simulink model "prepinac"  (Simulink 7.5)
settings: Solver=ode45  StartTime=0.0  StopTime=20  FixedStep=1  MaxStep=1  RelTol=1e-3
libraries: commutil2 x32, dspmtrx3 x28, simulink x20
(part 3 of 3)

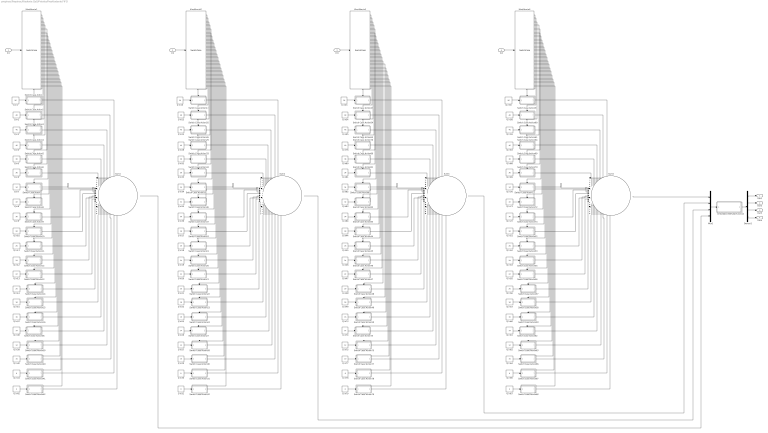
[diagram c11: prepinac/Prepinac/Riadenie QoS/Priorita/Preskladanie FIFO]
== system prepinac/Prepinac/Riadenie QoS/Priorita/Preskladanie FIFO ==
  In1 : Inport  OutDataType=sfix(16)  OutScaling=2^0
  In2 : Inport  Port=2  OutDataType=sfix(16)  OutScaling=2^0
  In3 : Inport  Port=3  OutDataType=sfix(16)  OutScaling=2^0
  In4 : Inport  Port=4  OutDataType=sfix(16)  OutScaling=2^0
  "     Embedded MATLAB Function" : Stateflow chart  TreatAsAtomicUnit=on
  Demux1 : Demux
  Klasifikacia{1..4} (4 alike) : SwitchCase  CaseConditions={0,8,10,12,14,16,18,20,22,24,26,28,30,32,34,36,38,40,46,48,56}  ShowDefaultCase=off
  Mux1 : Mux
  Q in{1,16,43,50} (4 alike) : Constant  Value=56  VectorParams1D=off  OutDataTypeMode=double  OutDataType=sfix(16)  OutScaling=2^0  OutDataTypeStr=double  SampleTime=-1
  Q in{10,17,44,51} (4 alike) : Constant  Value=28  VectorParams1D=off  OutDataTypeMode=double  OutDataType=sfix(16)  OutScaling=2^0  OutDataTypeStr=double  SampleTime=-1
  Q in{11,18,45,52} (4 alike) : Constant  Value=26  VectorParams1D=off  OutDataTypeMode=double  OutDataType=sfix(16)  OutScaling=2^0  OutDataTypeStr=double  SampleTime=-1
  Q in{12,19,46,53} (4 alike) : Constant  Value=24  VectorParams1D=off  OutDataTypeMode=double  OutDataType=sfix(16)  OutScaling=2^0  OutDataTypeStr=double  SampleTime=-1
  Q in{13,20,47,55} (4 alike) : Constant  Value=22  VectorParams1D=off  OutDataTypeMode=double  OutDataType=sfix(16)  OutScaling=2^0  OutDataTypeStr=double  SampleTime=-1
  Q in{14,21,48,56} (4 alike) : Constant  Value=20  VectorParams1D=off  OutDataTypeMode=double  OutDataType=sfix(16)  OutScaling=2^0  OutDataTypeStr=double  SampleTime=-1
  Q in{15,22,49,57} (4 alike) : Constant  Value=18  VectorParams1D=off  OutDataTypeMode=double  OutDataType=sfix(16)  OutScaling=2^0  OutDataTypeStr=double  SampleTime=-1
  Q in{2,23,54,58} (4 alike) : Constant  Value=48  VectorParams1D=off  OutDataTypeMode=double  OutDataType=sfix(16)  OutScaling=2^0  OutDataTypeStr=double  SampleTime=-1
  Q in{3,24,59,65} (4 alike) : Constant  Value=46  VectorParams1D=off  OutDataTypeMode=double  OutDataType=sfix(16)  OutScaling=2^0  OutDataTypeStr=double  SampleTime=-1
  Q in{25,37,60,73} (4 alike) : Constant  Value=16  VectorParams1D=off  OutDataTypeMode=double  OutDataType=sfix(16)  OutScaling=2^0  OutDataTypeStr=double  SampleTime=-1
  Q in{26,38,61,74} (4 alike) : Constant  Value=14  VectorParams1D=off  OutDataTypeMode=double  OutDataType=sfix(16)  OutScaling=2^0  OutDataTypeStr=double  SampleTime=-1
  Q in{27,39,62,75} (4 alike) : Constant  Value=12  VectorParams1D=off  OutDataTypeMode=double  OutDataType=sfix(16)  OutScaling=2^0  OutDataTypeStr=double  SampleTime=-1
  Q in{4,28,63,76} (4 alike) : Constant  Value=40  VectorParams1D=off  OutDataTypeMode=double  OutDataType=sfix(16)  OutScaling=2^0  OutDataTypeStr=double  SampleTime=-1
  Q in{29,40,64,77} (4 alike) : Constant  Value=10  VectorParams1D=off  OutDataTypeMode=double  OutDataType=sfix(16)  OutScaling=2^0  OutDataTypeStr=double  SampleTime=-1
  Q in{30,41,66,78} (4 alike) : Constant  Value=8  VectorParams1D=off  OutDataTypeMode=double  OutDataType=sfix(16)  OutScaling=2^0  OutDataTypeStr=double  SampleTime=-1
  Q in{31,42,67,79} (4 alike) : Constant  Value=0  VectorParams1D=off  OutDataTypeMode=double  OutDataType=sfix(16)  OutScaling=2^0  OutDataTypeStr=double  SampleTime=-1
  Q in{5,32,68,80} (4 alike) : Constant  Value=38  VectorParams1D=off  OutDataTypeMode=double  OutDataType=sfix(16)  OutScaling=2^0  OutDataTypeStr=double  SampleTime=-1
  Q in{6,33,69,81} (4 alike) : Constant  Value=36  VectorParams1D=off  OutDataTypeMode=double  OutDataType=sfix(16)  OutScaling=2^0  OutDataTypeStr=double  SampleTime=-1
  Q in{7,34,70,82} (4 alike) : Constant  Value=34  VectorParams1D=off  OutDataTypeMode=double  OutDataType=sfix(16)  OutScaling=2^0  OutDataTypeStr=double  SampleTime=-1
  Q in{8,35,71,83} (4 alike) : Constant  Value=32  VectorParams1D=off  OutDataTypeMode=double  OutDataType=sfix(16)  OutScaling=2^0  OutDataTypeStr=double  SampleTime=-1
  Q in{9,36,72,84} (4 alike) : Constant  Value=30  VectorParams1D=off  OutDataTypeMode=double  OutDataType=sfix(16)  OutScaling=2^0  OutDataTypeStr=double  SampleTime=-1
  Sum{1..4} (4 alike) : Sum  Inputs=|+++++++++++++++++++++  OutDataType=sfix(16)  OutScaling=2^0
  Switch Case Action1 : Subsystem  TreatAsAtomicUnit=on
  Switch Case Action10 : Subsystem  TreatAsAtomicUnit=on
  Switch Case Action11 : Subsystem  TreatAsAtomicUnit=on
  Switch Case Action12 : Subsystem  TreatAsAtomicUnit=on
  Switch Case Action13 : Subsystem  TreatAsAtomicUnit=on
  Switch Case Action14 : Subsystem  TreatAsAtomicUnit=on
  Switch Case Action15 : Subsystem  TreatAsAtomicUnit=on
  Switch Case Action16 : Subsystem  TreatAsAtomicUnit=on
  Switch Case Action17 : Subsystem  TreatAsAtomicUnit=on
  Switch Case Action18 : Subsystem  TreatAsAtomicUnit=on
  Switch Case Action19 : Subsystem  TreatAsAtomicUnit=on
  Switch Case Action2 : Subsystem  TreatAsAtomicUnit=on
  Switch Case Action20 : Subsystem  TreatAsAtomicUnit=on
  Switch Case Action21 : Subsystem  TreatAsAtomicUnit=on
  Switch Case Action22 : Subsystem  TreatAsAtomicUnit=on
  Switch Case Action23 : Subsystem  TreatAsAtomicUnit=on
  Switch Case Action24 : Subsystem  TreatAsAtomicUnit=on
  Switch Case Action25 : Subsystem  TreatAsAtomicUnit=on
  Switch Case Action26 : Subsystem  TreatAsAtomicUnit=on
  Switch Case Action27 : Subsystem  TreatAsAtomicUnit=on
  Switch Case Action28 : Subsystem  TreatAsAtomicUnit=on
  Switch Case Action29 : Subsystem  TreatAsAtomicUnit=on
  Switch Case Action3 : Subsystem  TreatAsAtomicUnit=on
  Switch Case Action30 : Subsystem  TreatAsAtomicUnit=on
  Switch Case Action31 : Subsystem  TreatAsAtomicUnit=on
  Switch Case Action32 : Subsystem  TreatAsAtomicUnit=on
  Switch Case Action33 : Subsystem  TreatAsAtomicUnit=on
  Switch Case Action34 : Subsystem  TreatAsAtomicUnit=on
  Switch Case Action35 : Subsystem  TreatAsAtomicUnit=on
  Switch Case Action36 : Subsystem  TreatAsAtomicUnit=on
  Switch Case Action37 : Subsystem  TreatAsAtomicUnit=on
  Switch Case Action38 : Subsystem  TreatAsAtomicUnit=on
  Switch Case Action39 : Subsystem  TreatAsAtomicUnit=on
  Switch Case Action4 : Subsystem  TreatAsAtomicUnit=on
  Switch Case Action40 : Subsystem  TreatAsAtomicUnit=on
  Switch Case Action41 : Subsystem  TreatAsAtomicUnit=on
  Switch Case Action42 : Subsystem  TreatAsAtomicUnit=on
  Switch Case Action43 : Subsystem  TreatAsAtomicUnit=on
  Switch Case Action44 : Subsystem  TreatAsAtomicUnit=on
  Switch Case Action45 : Subsystem  TreatAsAtomicUnit=on
  Switch Case Action46 : Subsystem  TreatAsAtomicUnit=on
  Switch Case Action47 : Subsystem  TreatAsAtomicUnit=on
  Switch Case Action48 : Subsystem  TreatAsAtomicUnit=on
  Switch Case Action49 : Subsystem  TreatAsAtomicUnit=on
  Switch Case Action5 : Subsystem  TreatAsAtomicUnit=on
  Switch Case Action50 : Subsystem  TreatAsAtomicUnit=on
  Switch Case Action51 : Subsystem  TreatAsAtomicUnit=on
  Switch Case Action52 : Subsystem  TreatAsAtomicUnit=on
  Switch Case Action53 : Subsystem  TreatAsAtomicUnit=on
  Switch Case Action54 : Subsystem  TreatAsAtomicUnit=on
  Switch Case Action55 : Subsystem  TreatAsAtomicUnit=on
  Switch Case Action56 : Subsystem  TreatAsAtomicUnit=on
  Switch Case Action57 : Subsystem  TreatAsAtomicUnit=on
  Switch Case Action58 : Subsystem  TreatAsAtomicUnit=on
  Switch Case Action59 : Subsystem  TreatAsAtomicUnit=on
  Switch Case Action6 : Subsystem  TreatAsAtomicUnit=on
  Switch Case Action60 : Subsystem  TreatAsAtomicUnit=on
  Switch Case Action61 : Subsystem  TreatAsAtomicUnit=on
  Switch Case Action62 : Subsystem  TreatAsAtomicUnit=on
  Switch Case Action63 : Subsystem  TreatAsAtomicUnit=on
  Switch Case Action64 : Subsystem  TreatAsAtomicUnit=on
  Switch Case Action65 : Subsystem  TreatAsAtomicUnit=on
  Switch Case Action66 : Subsystem  TreatAsAtomicUnit=on
  Switch Case Action67 : Subsystem  TreatAsAtomicUnit=on
  Switch Case Action68 : Subsystem  TreatAsAtomicUnit=on
  Switch Case Action69 : Subsystem  TreatAsAtomicUnit=on
  Switch Case Action7 : Subsystem  TreatAsAtomicUnit=on
  Switch Case Action70 : Subsystem  TreatAsAtomicUnit=on
  Switch Case Action71 : Subsystem  TreatAsAtomicUnit=on
  Switch Case Action72 : Subsystem  TreatAsAtomicUnit=on
  Switch Case Action73 : Subsystem  TreatAsAtomicUnit=on
  Switch Case Action74 : Subsystem  TreatAsAtomicUnit=on
  Switch Case Action75 : Subsystem  TreatAsAtomicUnit=on
  Switch Case Action76 : Subsystem  TreatAsAtomicUnit=on
  Switch Case Action77 : Subsystem  TreatAsAtomicUnit=on
  Switch Case Action78 : Subsystem  TreatAsAtomicUnit=on
  Switch Case Action79 : Subsystem  TreatAsAtomicUnit=on
  Switch Case Action8 : Subsystem  TreatAsAtomicUnit=on
  Switch Case Action80 : Subsystem  TreatAsAtomicUnit=on
  Switch Case Action81 : Subsystem  TreatAsAtomicUnit=on
  Switch Case Action82 : Subsystem  TreatAsAtomicUnit=on
  Switch Case Action83 : Subsystem  TreatAsAtomicUnit=on
  Switch Case Action84 : Subsystem  TreatAsAtomicUnit=on
  Switch Case Action9 : Subsystem  TreatAsAtomicUnit=on
  Out1 : Outport  OutDataType=sfix(16)  OutScaling=2^0
  Out2 : Outport  Port=2  OutDataType=sfix(16)  OutScaling=2^0
  Out3 : Outport  Port=3  OutDataType=sfix(16)  OutScaling=2^0
  Out4 : Outport  Port=4  OutDataType=sfix(16)  OutScaling=2^0
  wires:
  Mux1/1 -> "     Embedded MATLAB Function"/1(x)
  "     Embedded MATLAB Function"/1(y) -> Demux1/1
  Demux1/1 -> Out1/1
  Demux1/2 -> Out2/1
  Demux1/3 -> Out3/1
  Demux1/4 -> Out4/1
  Switch Case Action1/1(Out1) -> Sum1/1
  Switch Case Action2/1(Out1) -> Sum1/2
  Switch Case Action3/1(Out1) -> Sum1/3
  Switch Case Action4/1(Out1) -> Sum1/4
  Q in1/1 -> Switch Case Action1/1(In1)
  Q in2/1 -> Switch Case Action2/1(In1)
  Q in3/1 -> Switch Case Action3/1(In1)
  Q in4/1 -> Switch Case Action4/1(In1)
  Q in5/1 -> Switch Case Action5/1(In1)
  Q in6/1 -> Switch Case Action6/1(In1)
  Q in7/1 -> Switch Case Action7/1(In1)
  Q in8/1 -> Switch Case Action8/1(In1)
  Q in9/1 -> Switch Case Action9/1(In1)
  Q in10/1 -> Switch Case Action10/1(In1)
  Q in11/1 -> Switch Case Action11/1(In1)
  Q in12/1 -> Switch Case Action12/1(In1)
  Q in13/1 -> Switch Case Action13/1(In1)
  Q in14/1 -> Switch Case Action14/1(In1)
  Q in15/1 -> Switch Case Action15/1(In1)
  Q in37/1 -> Switch Case Action16/1(In1)
  Q in38/1 -> Switch Case Action38/1(In1)
  Q in39/1 -> Switch Case Action39/1(In1)
  Q in40/1 -> Switch Case Action40/1(In1)
  Q in41/1 -> Switch Case Action41/1(In1)
  Q in42/1 -> Switch Case Action42/1(In1)
  Switch Case Action5/1(Out1) -> Sum1/5
  Switch Case Action6/1(Out1) -> Sum1/6
  Switch Case Action7/1(Out1) -> Sum1/7
  Switch Case Action8/1(Out1) -> Sum1/8
  Switch Case Action42/1(Out1) -> Sum1/21
  Switch Case Action41/1(Out1) -> Sum1/20
  Switch Case Action40/1(Out1) -> Sum1/19
  Switch Case Action39/1(Out1) -> Sum1/18
  Switch Case Action38/1(Out1) -> Sum1/17
  Switch Case Action16/1(Out1) -> Sum1/16
  Switch Case Action15/1(Out1) -> Sum1/15
  Switch Case Action14/1(Out1) -> Sum1/14
  Switch Case Action13/1(Out1) -> Sum1/13
  Switch Case Action12/1(Out1) -> Sum1/12
  Switch Case Action11/1(Out1) -> Sum1/11
  Switch Case Action10/1(Out1) -> Sum1/10
  Switch Case Action9/1(Out1) -> Sum1/9
  Sum1/1 -> Mux1/4
  In1/1 -> Klasifikacia1/1
  Klasifikacia1/1 -> Switch Case Action1/Action
  Klasifikacia1/2 -> Switch Case Action2/Action
  Klasifikacia1/3 -> Switch Case Action3/Action
  Klasifikacia1/4 -> Switch Case Action4/Action
  Klasifikacia1/5 -> Switch Case Action5/Action
  Klasifikacia1/6 -> Switch Case Action6/Action
  Klasifikacia1/7 -> Switch Case Action7/Action
  Klasifikacia1/8 -> Switch Case Action8/Action
  Klasifikacia1/9 -> Switch Case Action9/Action
  Klasifikacia1/10 -> Switch Case Action10/Action
  Klasifikacia1/11 -> Switch Case Action11/Action
  Klasifikacia1/12 -> Switch Case Action12/Action
  Klasifikacia1/13 -> Switch Case Action13/Action
  Klasifikacia1/14 -> Switch Case Action14/Action
  Klasifikacia1/15 -> Switch Case Action15/Action
  Klasifikacia1/16 -> Switch Case Action16/Action
  Klasifikacia1/17 -> Switch Case Action38/Action
  Klasifikacia1/18 -> Switch Case Action39/Action
  Klasifikacia1/19 -> Switch Case Action40/Action
  Klasifikacia1/20 -> Switch Case Action41/Action
  Klasifikacia1/21 -> Switch Case Action42/Action
  Switch Case Action17/1(Out1) -> Sum2/1
  Switch Case Action25/1(Out1) -> Sum2/2
  Switch Case Action26/1(Out1) -> Sum2/3
  Switch Case Action29/1(Out1) -> Sum2/4
  Q in16/1 -> Switch Case Action17/1(In1)
  Q in23/1 -> Switch Case Action25/1(In1)
  Q in24/1 -> Switch Case Action26/1(In1)
  Q in28/1 -> Switch Case Action29/1(In1)
  Q in32/1 -> Switch Case Action33/1(In1)
  Q in33/1 -> Switch Case Action34/1(In1)
  Q in34/1 -> Switch Case Action35/1(In1)
  Q in35/1 -> Switch Case Action36/1(In1)
  Q in36/1 -> Switch Case Action37/1(In1)
  Q in17/1 -> Switch Case Action18/1(In1)
  Q in18/1 -> Switch Case Action19/1(In1)
  Q in19/1 -> Switch Case Action20/1(In1)
  Q in20/1 -> Switch Case Action21/1(In1)
  Q in21/1 -> Switch Case Action22/1(In1)
  Q in22/1 -> Switch Case Action23/1(In1)
  Q in25/1 -> Switch Case Action24/1(In1)
  Q in26/1 -> Switch Case Action27/1(In1)
  Q in27/1 -> Switch Case Action28/1(In1)
  Q in29/1 -> Switch Case Action30/1(In1)
  Q in30/1 -> Switch Case Action31/1(In1)
  Q in31/1 -> Switch Case Action32/1(In1)
  Switch Case Action33/1(Out1) -> Sum2/5
  Switch Case Action34/1(Out1) -> Sum2/6
  Switch Case Action35/1(Out1) -> Sum2/7
  Switch Case Action36/1(Out1) -> Sum2/8
  Switch Case Action32/1(Out1) -> Sum2/21
  Switch Case Action31/1(Out1) -> Sum2/20
  Switch Case Action30/1(Out1) -> Sum2/19
  Switch Case Action28/1(Out1) -> Sum2/18
  Switch Case Action27/1(Out1) -> Sum2/17
  Switch Case Action24/1(Out1) -> Sum2/16
  Switch Case Action23/1(Out1) -> Sum2/15
  Switch Case Action22/1(Out1) -> Sum2/14
  Switch Case Action21/1(Out1) -> Sum2/13
  Switch Case Action20/1(Out1) -> Sum2/12
  Switch Case Action19/1(Out1) -> Sum2/11
  Switch Case Action18/1(Out1) -> Sum2/10
  Switch Case Action37/1(Out1) -> Sum2/9
  In2/1 -> Klasifikacia2/1
  Klasifikacia2/1 -> Switch Case Action17/Action
  Klasifikacia2/2 -> Switch Case Action25/Action
  Klasifikacia2/3 -> Switch Case Action26/Action
  Klasifikacia2/4 -> Switch Case Action29/Action
  Klasifikacia2/5 -> Switch Case Action33/Action
  Klasifikacia2/6 -> Switch Case Action34/Action
  Klasifikacia2/7 -> Switch Case Action35/Action
  Klasifikacia2/8 -> Switch Case Action36/Action
  Klasifikacia2/9 -> Switch Case Action37/Action
  Klasifikacia2/10 -> Switch Case Action18/Action
  Klasifikacia2/11 -> Switch Case Action19/Action
  Klasifikacia2/12 -> Switch Case Action20/Action
  Klasifikacia2/13 -> Switch Case Action21/Action
  Klasifikacia2/14 -> Switch Case Action22/Action
  Klasifikacia2/15 -> Switch Case Action23/Action
  Klasifikacia2/16 -> Switch Case Action24/Action
  Klasifikacia2/17 -> Switch Case Action27/Action
  Klasifikacia2/18 -> Switch Case Action28/Action
  Klasifikacia2/19 -> Switch Case Action30/Action
  Klasifikacia2/20 -> Switch Case Action31/Action
  Klasifikacia2/21 -> Switch Case Action32/Action
  Switch Case Action43/1(Out1) -> Sum3/1
  Switch Case Action54/1(Out1) -> Sum3/2
  Switch Case Action65/1(Out1) -> Sum3/3
  Switch Case Action76/1(Out1) -> Sum3/4
  Q in43/1 -> Switch Case Action43/1(In1)
  Q in54/1 -> Switch Case Action54/1(In1)
  Q in65/1 -> Switch Case Action65/1(In1)
  Q in76/1 -> Switch Case Action76/1(In1)
  Q in80/1 -> Switch Case Action80/1(In1)
  Q in81/1 -> Switch Case Action81/1(In1)
  Q in82/1 -> Switch Case Action82/1(In1)
  Q in83/1 -> Switch Case Action83/1(In1)
  Q in84/1 -> Switch Case Action84/1(In1)
  Q in44/1 -> Switch Case Action44/1(In1)
  Q in45/1 -> Switch Case Action45/1(In1)
  Q in46/1 -> Switch Case Action46/1(In1)
  Q in47/1 -> Switch Case Action47/1(In1)
  Q in48/1 -> Switch Case Action48/1(In1)
  Q in49/1 -> Switch Case Action49/1(In1)
  Q in73/1 -> Switch Case Action50/1(In1)
  Q in74/1 -> Switch Case Action74/1(In1)
  Q in75/1 -> Switch Case Action75/1(In1)
  Q in77/1 -> Switch Case Action77/1(In1)
  Q in78/1 -> Switch Case Action78/1(In1)
  Q in79/1 -> Switch Case Action79/1(In1)
  Switch Case Action80/1(Out1) -> Sum3/5
  Switch Case Action81/1(Out1) -> Sum3/6
  Switch Case Action82/1(Out1) -> Sum3/7
  Switch Case Action83/1(Out1) -> Sum3/8
  Switch Case Action79/1(Out1) -> Sum3/21
  Switch Case Action78/1(Out1) -> Sum3/20
  Switch Case Action77/1(Out1) -> Sum3/19
  Switch Case Action75/1(Out1) -> Sum3/18
  Switch Case Action74/1(Out1) -> Sum3/17
  Switch Case Action50/1(Out1) -> Sum3/16
  Switch Case Action49/1(Out1) -> Sum3/15
  Switch Case Action48/1(Out1) -> Sum3/14
  Switch Case Action47/1(Out1) -> Sum3/13
  Switch Case Action46/1(Out1) -> Sum3/12
  Switch Case Action45/1(Out1) -> Sum3/11
  Switch Case Action44/1(Out1) -> Sum3/10
  Switch Case Action84/1(Out1) -> Sum3/9
  In3/1 -> Klasifikacia3/1
  Klasifikacia3/1 -> Switch Case Action43/Action
  Klasifikacia3/2 -> Switch Case Action54/Action
  Klasifikacia3/3 -> Switch Case Action65/Action
  Klasifikacia3/4 -> Switch Case Action76/Action
  Klasifikacia3/5 -> Switch Case Action80/Action
  Klasifikacia3/6 -> Switch Case Action81/Action
  Klasifikacia3/7 -> Switch Case Action82/Action
  Klasifikacia3/8 -> Switch Case Action83/Action
  Klasifikacia3/9 -> Switch Case Action84/Action
  Klasifikacia3/10 -> Switch Case Action44/Action
  Klasifikacia3/11 -> Switch Case Action45/Action
  Klasifikacia3/12 -> Switch Case Action46/Action
  Klasifikacia3/13 -> Switch Case Action47/Action
  Klasifikacia3/14 -> Switch Case Action48/Action
  Klasifikacia3/15 -> Switch Case Action49/Action
  Klasifikacia3/16 -> Switch Case Action50/Action
  Klasifikacia3/17 -> Switch Case Action74/Action
  Klasifikacia3/18 -> Switch Case Action75/Action
  Klasifikacia3/19 -> Switch Case Action77/Action
  Klasifikacia3/20 -> Switch Case Action78/Action
  Klasifikacia3/21 -> Switch Case Action79/Action
  Switch Case Action51/1(Out1) -> Sum4/1
  Switch Case Action60/1(Out1) -> Sum4/2
  Switch Case Action61/1(Out1) -> Sum4/3
  Switch Case Action64/1(Out1) -> Sum4/4
  Q in50/1 -> Switch Case Action51/1(In1)
  Q in58/1 -> Switch Case Action60/1(In1)
  Q in59/1 -> Switch Case Action61/1(In1)
  Q in63/1 -> Switch Case Action64/1(In1)
  Q in68/1 -> Switch Case Action69/1(In1)
  Q in69/1 -> Switch Case Action70/1(In1)
  Q in70/1 -> Switch Case Action71/1(In1)
  Q in71/1 -> Switch Case Action72/1(In1)
  Q in72/1 -> Switch Case Action73/1(In1)
  Q in51/1 -> Switch Case Action52/1(In1)
  Q in52/1 -> Switch Case Action53/1(In1)
  Q in53/1 -> Switch Case Action55/1(In1)
  Q in55/1 -> Switch Case Action56/1(In1)
  Q in56/1 -> Switch Case Action57/1(In1)
  Q in57/1 -> Switch Case Action58/1(In1)
  Q in60/1 -> Switch Case Action59/1(In1)
  Q in61/1 -> Switch Case Action62/1(In1)
  Q in62/1 -> Switch Case Action63/1(In1)
  Q in64/1 -> Switch Case Action66/1(In1)
  Q in66/1 -> Switch Case Action67/1(In1)
  Q in67/1 -> Switch Case Action68/1(In1)
  Switch Case Action69/1(Out1) -> Sum4/5
  Switch Case Action70/1(Out1) -> Sum4/6
  Switch Case Action71/1(Out1) -> Sum4/7
  Switch Case Action72/1(Out1) -> Sum4/8
  Switch Case Action68/1(Out1) -> Sum4/21
  Switch Case Action67/1(Out1) -> Sum4/20
  Switch Case Action66/1(Out1) -> Sum4/19
  Switch Case Action63/1(Out1) -> Sum4/18
  Switch Case Action62/1(Out1) -> Sum4/17
  Switch Case Action59/1(Out1) -> Sum4/16
  Switch Case Action58/1(Out1) -> Sum4/15
  Switch Case Action57/1(Out1) -> Sum4/14
  Switch Case Action56/1(Out1) -> Sum4/13
  Switch Case Action55/1(Out1) -> Sum4/12
  Switch Case Action53/1(Out1) -> Sum4/11
  Switch Case Action52/1(Out1) -> Sum4/10
  Switch Case Action73/1(Out1) -> Sum4/9
  In4/1 -> Klasifikacia4/1
  Klasifikacia4/1 -> Switch Case Action51/Action
  Klasifikacia4/2 -> Switch Case Action60/Action
  Klasifikacia4/3 -> Switch Case Action61/Action
  Klasifikacia4/4 -> Switch Case Action64/Action
  Klasifikacia4/5 -> Switch Case Action69/Action
  Klasifikacia4/6 -> Switch Case Action70/Action
  Klasifikacia4/7 -> Switch Case Action71/Action
  Klasifikacia4/8 -> Switch Case Action72/Action
  Klasifikacia4/9 -> Switch Case Action73/Action
  Klasifikacia4/10 -> Switch Case Action52/Action
  Klasifikacia4/11 -> Switch Case Action53/Action
  Klasifikacia4/12 -> Switch Case Action55/Action
  Klasifikacia4/13 -> Switch Case Action56/Action
  Klasifikacia4/14 -> Switch Case Action57/Action
  Klasifikacia4/15 -> Switch Case Action58/Action
  Klasifikacia4/16 -> Switch Case Action59/Action
  Klasifikacia4/17 -> Switch Case Action62/Action
  Klasifikacia4/18 -> Switch Case Action63/Action
  Klasifikacia4/19 -> Switch Case Action66/Action
  Klasifikacia4/20 -> Switch Case Action67/Action
  Klasifikacia4/21 -> Switch Case Action68/Action
  Sum2/1 -> Mux1/3
  Sum3/1 -> Mux1/2
  Sum4/1 -> Mux1/1

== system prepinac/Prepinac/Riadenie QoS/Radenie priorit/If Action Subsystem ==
  In1 : Inport  OutDataType=sfix(16)  OutScaling=2^0
  Action Port : ActionPort  ActionType=then
  Out1 : Outport  OutDataType=sfix(16)  OutScaling=2^0
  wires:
  In1/1 -> Out1/1

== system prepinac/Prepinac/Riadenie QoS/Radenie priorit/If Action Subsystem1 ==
  In1 : Inport  OutDataType=sfix(16)  OutScaling=2^0
  Action Port : ActionPort  ActionType=elseif
  Out1 : Outport  OutDataType=sfix(16)  OutScaling=2^0
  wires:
  In1/1 -> Out1/1

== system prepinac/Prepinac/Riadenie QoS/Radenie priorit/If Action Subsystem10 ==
  In1 : Inport  OutDataType=sfix(16)  OutScaling=2^0
  Action Port : ActionPort  ActionType=then
  Out1 : Outport  OutDataType=sfix(16)  OutScaling=2^0
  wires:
  In1/1 -> Out1/1

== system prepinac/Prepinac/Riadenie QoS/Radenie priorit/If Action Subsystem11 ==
  In1 : Inport  OutDataType=sfix(16)  OutScaling=2^0
  Action Port : ActionPort  ActionType=elseif
  Out1 : Outport  OutDataType=sfix(16)  OutScaling=2^0
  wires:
  In1/1 -> Out1/1

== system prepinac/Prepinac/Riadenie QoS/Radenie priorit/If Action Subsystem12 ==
  In1 : Inport  OutDataType=sfix(16)  OutScaling=2^0
  Action Port : ActionPort  ActionType=then
  Out1 : Outport  OutDataType=sfix(16)  OutScaling=2^0
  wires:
  In1/1 -> Out1/1

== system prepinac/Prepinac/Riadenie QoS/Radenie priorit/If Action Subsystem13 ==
  In1 : Inport  OutDataType=sfix(16)  OutScaling=2^0
  Action Port : ActionPort  ActionType=elseif
  Out1 : Outport  OutDataType=sfix(16)  OutScaling=2^0
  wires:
  In1/1 -> Out1/1

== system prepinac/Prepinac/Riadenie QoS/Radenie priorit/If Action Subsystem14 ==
  In1 : Inport  OutDataType=sfix(16)  OutScaling=2^0
  Action Port : ActionPort  ActionType=then
  Out1 : Outport  OutDataType=sfix(16)  OutScaling=2^0
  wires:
  In1/1 -> Out1/1

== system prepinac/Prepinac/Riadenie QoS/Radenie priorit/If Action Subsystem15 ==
  In1 : Inport  OutDataType=sfix(16)  OutScaling=2^0
  Action Port : ActionPort  ActionType=elseif
  Out1 : Outport  OutDataType=sfix(16)  OutScaling=2^0
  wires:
  In1/1 -> Out1/1

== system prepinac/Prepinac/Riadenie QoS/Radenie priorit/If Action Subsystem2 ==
  In1 : Inport  OutDataType=sfix(16)  OutScaling=2^0
  Action Port : ActionPort  ActionType=then
  Out1 : Outport  OutDataType=sfix(16)  OutScaling=2^0
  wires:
  In1/1 -> Out1/1

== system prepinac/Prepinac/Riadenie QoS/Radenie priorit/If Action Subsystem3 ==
  In1 : Inport  OutDataType=sfix(16)  OutScaling=2^0
  Action Port : ActionPort  ActionType=elseif
  Out1 : Outport  OutDataType=sfix(16)  OutScaling=2^0
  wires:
  In1/1 -> Out1/1

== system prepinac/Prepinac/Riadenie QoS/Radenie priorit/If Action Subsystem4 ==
  In1 : Inport  OutDataType=sfix(16)  OutScaling=2^0
  Action Port : ActionPort  ActionType=then
  Out1 : Outport  OutDataType=sfix(16)  OutScaling=2^0
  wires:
  In1/1 -> Out1/1

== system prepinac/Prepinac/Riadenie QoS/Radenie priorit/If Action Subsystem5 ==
  In1 : Inport  OutDataType=sfix(16)  OutScaling=2^0
  Action Port : ActionPort  ActionType=elseif
  Out1 : Outport  OutDataType=sfix(16)  OutScaling=2^0
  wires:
  In1/1 -> Out1/1

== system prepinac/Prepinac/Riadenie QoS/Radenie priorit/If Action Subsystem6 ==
  In1 : Inport  OutDataType=sfix(16)  OutScaling=2^0
  Action Port : ActionPort  ActionType=then
  Out1 : Outport  OutDataType=sfix(16)  OutScaling=2^0
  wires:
  In1/1 -> Out1/1

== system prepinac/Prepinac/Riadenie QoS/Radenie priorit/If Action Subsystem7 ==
  In1 : Inport  OutDataType=sfix(16)  OutScaling=2^0
  Action Port : ActionPort  ActionType=elseif
  Out1 : Outport  OutDataType=sfix(16)  OutScaling=2^0
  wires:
  In1/1 -> Out1/1

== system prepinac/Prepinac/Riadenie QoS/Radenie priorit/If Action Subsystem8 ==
  In1 : Inport  OutDataType=sfix(16)  OutScaling=2^0
  Action Port : ActionPort  ActionType=then
  Out1 : Outport  OutDataType=sfix(16)  OutScaling=2^0
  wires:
  In1/1 -> Out1/1

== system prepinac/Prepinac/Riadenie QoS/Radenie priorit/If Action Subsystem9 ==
  In1 : Inport  OutDataType=sfix(16)  OutScaling=2^0
  Action Port : ActionPort  ActionType=elseif
  Out1 : Outport  OutDataType=sfix(16)  OutScaling=2^0
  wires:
  In1/1 -> Out1/1

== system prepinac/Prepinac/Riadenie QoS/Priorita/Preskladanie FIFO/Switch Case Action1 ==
  In1 : Inport  OutDataType=sfix(16)  OutScaling=2^0
  Action Port : ActionPort  ActionType=case
  Out1 : Outport  OutDataType=sfix(16)  OutScaling=2^0
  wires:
  In1/1 -> Out1/1

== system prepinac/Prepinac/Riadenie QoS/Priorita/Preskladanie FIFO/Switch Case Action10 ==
  In1 : Inport  OutDataType=sfix(16)  OutScaling=2^0
  Action Port : ActionPort  ActionType=case
  Out1 : Outport  OutDataType=sfix(16)  OutScaling=2^0
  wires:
  In1/1 -> Out1/1

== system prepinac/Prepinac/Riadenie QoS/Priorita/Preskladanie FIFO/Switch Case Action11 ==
  In1 : Inport  OutDataType=sfix(16)  OutScaling=2^0
  Action Port : ActionPort  ActionType=case
  Out1 : Outport  OutDataType=sfix(16)  OutScaling=2^0
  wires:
  In1/1 -> Out1/1

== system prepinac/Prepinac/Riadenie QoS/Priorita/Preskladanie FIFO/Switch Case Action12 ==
  In1 : Inport  OutDataType=sfix(16)  OutScaling=2^0
  Action Port : ActionPort  ActionType=case
  Out1 : Outport  OutDataType=sfix(16)  OutScaling=2^0
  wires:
  In1/1 -> Out1/1

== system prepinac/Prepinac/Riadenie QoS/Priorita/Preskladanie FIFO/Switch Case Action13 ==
  In1 : Inport  OutDataType=sfix(16)  OutScaling=2^0
  Action Port : ActionPort  ActionType=case
  Out1 : Outport  OutDataType=sfix(16)  OutScaling=2^0
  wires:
  In1/1 -> Out1/1

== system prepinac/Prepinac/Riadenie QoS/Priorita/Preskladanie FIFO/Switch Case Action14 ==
  In1 : Inport  OutDataType=sfix(16)  OutScaling=2^0
  Action Port : ActionPort  ActionType=case
  Out1 : Outport  OutDataType=sfix(16)  OutScaling=2^0
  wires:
  In1/1 -> Out1/1

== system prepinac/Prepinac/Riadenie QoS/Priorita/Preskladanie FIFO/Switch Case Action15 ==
  In1 : Inport  OutDataType=sfix(16)  OutScaling=2^0
  Action Port : ActionPort  ActionType=case
  Out1 : Outport  OutDataType=sfix(16)  OutScaling=2^0
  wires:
  In1/1 -> Out1/1

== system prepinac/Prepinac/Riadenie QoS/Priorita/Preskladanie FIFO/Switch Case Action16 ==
  In1 : Inport  OutDataType=sfix(16)  OutScaling=2^0
  Action Port : ActionPort  ActionType=case
  Out1 : Outport  OutDataType=sfix(16)  OutScaling=2^0
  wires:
  In1/1 -> Out1/1

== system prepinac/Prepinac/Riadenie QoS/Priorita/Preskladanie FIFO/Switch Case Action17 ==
  In1 : Inport  OutDataType=sfix(16)  OutScaling=2^0
  Action Port : ActionPort  ActionType=case
  Out1 : Outport  OutDataType=sfix(16)  OutScaling=2^0
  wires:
  In1/1 -> Out1/1

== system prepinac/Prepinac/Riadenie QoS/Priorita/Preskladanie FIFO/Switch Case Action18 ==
  In1 : Inport  OutDataType=sfix(16)  OutScaling=2^0
  Action Port : ActionPort  ActionType=case
  Out1 : Outport  OutDataType=sfix(16)  OutScaling=2^0
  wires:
  In1/1 -> Out1/1

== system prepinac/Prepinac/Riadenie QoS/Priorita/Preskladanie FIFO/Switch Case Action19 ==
  In1 : Inport  OutDataType=sfix(16)  OutScaling=2^0
  Action Port : ActionPort  ActionType=case
  Out1 : Outport  OutDataType=sfix(16)  OutScaling=2^0
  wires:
  In1/1 -> Out1/1

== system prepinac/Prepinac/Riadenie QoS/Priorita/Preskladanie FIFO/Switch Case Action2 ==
  In1 : Inport  OutDataType=sfix(16)  OutScaling=2^0
  Action Port : ActionPort  ActionType=case
  Out1 : Outport  OutDataType=sfix(16)  OutScaling=2^0
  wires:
  In1/1 -> Out1/1

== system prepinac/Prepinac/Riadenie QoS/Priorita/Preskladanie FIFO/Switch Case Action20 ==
  In1 : Inport  OutDataType=sfix(16)  OutScaling=2^0
  Action Port : ActionPort  ActionType=case
  Out1 : Outport  OutDataType=sfix(16)  OutScaling=2^0
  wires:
  In1/1 -> Out1/1

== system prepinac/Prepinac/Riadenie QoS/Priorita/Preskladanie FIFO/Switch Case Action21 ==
  In1 : Inport  OutDataType=sfix(16)  OutScaling=2^0
  Action Port : ActionPort  ActionType=case
  Out1 : Outport  OutDataType=sfix(16)  OutScaling=2^0
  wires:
  In1/1 -> Out1/1

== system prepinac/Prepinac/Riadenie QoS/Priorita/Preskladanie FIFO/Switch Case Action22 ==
  In1 : Inport  OutDataType=sfix(16)  OutScaling=2^0
  Action Port : ActionPort  ActionType=case
  Out1 : Outport  OutDataType=sfix(16)  OutScaling=2^0
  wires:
  In1/1 -> Out1/1

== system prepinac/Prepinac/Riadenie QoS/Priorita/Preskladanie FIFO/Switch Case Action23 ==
  In1 : Inport  OutDataType=sfix(16)  OutScaling=2^0
  Action Port : ActionPort  ActionType=case
  Out1 : Outport  OutDataType=sfix(16)  OutScaling=2^0
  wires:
  In1/1 -> Out1/1

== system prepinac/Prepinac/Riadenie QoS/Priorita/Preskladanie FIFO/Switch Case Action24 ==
  In1 : Inport  OutDataType=sfix(16)  OutScaling=2^0
  Action Port : ActionPort  ActionType=case
  Out1 : Outport  OutDataType=sfix(16)  OutScaling=2^0
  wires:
  In1/1 -> Out1/1

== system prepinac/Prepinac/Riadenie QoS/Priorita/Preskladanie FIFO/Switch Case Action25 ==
  In1 : Inport  OutDataType=sfix(16)  OutScaling=2^0
  Action Port : ActionPort  ActionType=case
  Out1 : Outport  OutDataType=sfix(16)  OutScaling=2^0
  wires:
  In1/1 -> Out1/1

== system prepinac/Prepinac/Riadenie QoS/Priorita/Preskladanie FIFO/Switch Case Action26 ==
  In1 : Inport  OutDataType=sfix(16)  OutScaling=2^0
  Action Port : ActionPort  ActionType=case
  Out1 : Outport  OutDataType=sfix(16)  OutScaling=2^0
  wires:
  In1/1 -> Out1/1

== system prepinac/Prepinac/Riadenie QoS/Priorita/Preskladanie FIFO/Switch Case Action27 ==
  In1 : Inport  OutDataType=sfix(16)  OutScaling=2^0
  Action Port : ActionPort  ActionType=case
  Out1 : Outport  OutDataType=sfix(16)  OutScaling=2^0
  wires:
  In1/1 -> Out1/1

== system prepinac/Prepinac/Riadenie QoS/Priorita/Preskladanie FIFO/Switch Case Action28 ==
  In1 : Inport  OutDataType=sfix(16)  OutScaling=2^0
  Action Port : ActionPort  ActionType=case
  Out1 : Outport  OutDataType=sfix(16)  OutScaling=2^0
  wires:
  In1/1 -> Out1/1

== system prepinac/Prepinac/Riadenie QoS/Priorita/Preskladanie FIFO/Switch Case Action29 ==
  In1 : Inport  OutDataType=sfix(16)  OutScaling=2^0
  Action Port : ActionPort  ActionType=case
  Out1 : Outport  OutDataType=sfix(16)  OutScaling=2^0
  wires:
  In1/1 -> Out1/1

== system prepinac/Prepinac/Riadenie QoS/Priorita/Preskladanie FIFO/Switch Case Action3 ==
  In1 : Inport  OutDataType=sfix(16)  OutScaling=2^0
  Action Port : ActionPort  ActionType=case
  Out1 : Outport  OutDataType=sfix(16)  OutScaling=2^0
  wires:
  In1/1 -> Out1/1

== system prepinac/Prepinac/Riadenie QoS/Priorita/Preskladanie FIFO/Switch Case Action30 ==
  In1 : Inport  OutDataType=sfix(16)  OutScaling=2^0
  Action Port : ActionPort  ActionType=case
  Out1 : Outport  OutDataType=sfix(16)  OutScaling=2^0
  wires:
  In1/1 -> Out1/1

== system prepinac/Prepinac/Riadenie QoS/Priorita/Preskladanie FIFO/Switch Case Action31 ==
  In1 : Inport  OutDataType=sfix(16)  OutScaling=2^0
  Action Port : ActionPort  ActionType=case
  Out1 : Outport  OutDataType=sfix(16)  OutScaling=2^0
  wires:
  In1/1 -> Out1/1

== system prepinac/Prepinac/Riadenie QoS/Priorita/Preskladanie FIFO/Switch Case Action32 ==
  In1 : Inport  OutDataType=sfix(16)  OutScaling=2^0
  Action Port : ActionPort  ActionType=case
  Out1 : Outport  OutDataType=sfix(16)  OutScaling=2^0
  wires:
  In1/1 -> Out1/1

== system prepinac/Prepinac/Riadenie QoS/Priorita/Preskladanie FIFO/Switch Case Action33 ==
  In1 : Inport  OutDataType=sfix(16)  OutScaling=2^0
  Action Port : ActionPort  ActionType=case
  Out1 : Outport  OutDataType=sfix(16)  OutScaling=2^0
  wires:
  In1/1 -> Out1/1

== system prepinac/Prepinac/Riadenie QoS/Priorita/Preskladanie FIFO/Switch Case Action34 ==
  In1 : Inport  OutDataType=sfix(16)  OutScaling=2^0
  Action Port : ActionPort  ActionType=case
  Out1 : Outport  OutDataType=sfix(16)  OutScaling=2^0
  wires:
  In1/1 -> Out1/1

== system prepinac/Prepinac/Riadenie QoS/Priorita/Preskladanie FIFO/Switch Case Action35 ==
  In1 : Inport  OutDataType=sfix(16)  OutScaling=2^0
  Action Port : ActionPort  ActionType=case
  Out1 : Outport  OutDataType=sfix(16)  OutScaling=2^0
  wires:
  In1/1 -> Out1/1

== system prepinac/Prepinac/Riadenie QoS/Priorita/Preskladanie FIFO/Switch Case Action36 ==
  In1 : Inport  OutDataType=sfix(16)  OutScaling=2^0
  Action Port : ActionPort  ActionType=case
  Out1 : Outport  OutDataType=sfix(16)  OutScaling=2^0
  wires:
  In1/1 -> Out1/1

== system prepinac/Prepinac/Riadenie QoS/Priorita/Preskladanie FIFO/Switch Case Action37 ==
  In1 : Inport  OutDataType=sfix(16)  OutScaling=2^0
  Action Port : ActionPort  ActionType=case
  Out1 : Outport  OutDataType=sfix(16)  OutScaling=2^0
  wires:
  In1/1 -> Out1/1

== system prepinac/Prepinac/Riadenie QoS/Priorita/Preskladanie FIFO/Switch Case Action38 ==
  In1 : Inport  OutDataType=sfix(16)  OutScaling=2^0
  Action Port : ActionPort  ActionType=case
  Out1 : Outport  OutDataType=sfix(16)  OutScaling=2^0
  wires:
  In1/1 -> Out1/1

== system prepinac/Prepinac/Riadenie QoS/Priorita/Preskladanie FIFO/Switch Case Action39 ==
  In1 : Inport  OutDataType=sfix(16)  OutScaling=2^0
  Action Port : ActionPort  ActionType=case
  Out1 : Outport  OutDataType=sfix(16)  OutScaling=2^0
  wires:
  In1/1 -> Out1/1

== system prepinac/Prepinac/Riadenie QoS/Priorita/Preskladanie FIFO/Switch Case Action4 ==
  In1 : Inport  OutDataType=sfix(16)  OutScaling=2^0
  Action Port : ActionPort  ActionType=case
  Out1 : Outport  OutDataType=sfix(16)  OutScaling=2^0
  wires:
  In1/1 -> Out1/1

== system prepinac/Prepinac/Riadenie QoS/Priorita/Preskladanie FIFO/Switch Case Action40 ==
  In1 : Inport  OutDataType=sfix(16)  OutScaling=2^0
  Action Port : ActionPort  ActionType=case
  Out1 : Outport  OutDataType=sfix(16)  OutScaling=2^0
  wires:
  In1/1 -> Out1/1

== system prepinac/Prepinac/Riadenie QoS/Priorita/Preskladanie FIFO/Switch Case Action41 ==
  In1 : Inport  OutDataType=sfix(16)  OutScaling=2^0
  Action Port : ActionPort  ActionType=case
  Out1 : Outport  OutDataType=sfix(16)  OutScaling=2^0
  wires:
  In1/1 -> Out1/1

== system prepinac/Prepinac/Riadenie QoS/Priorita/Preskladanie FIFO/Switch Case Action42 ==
  In1 : Inport  OutDataType=sfix(16)  OutScaling=2^0
  Action Port : ActionPort  ActionType=case
  Out1 : Outport  OutDataType=sfix(16)  OutScaling=2^0
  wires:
  In1/1 -> Out1/1

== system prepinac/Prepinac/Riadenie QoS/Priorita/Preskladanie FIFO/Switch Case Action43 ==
  In1 : Inport  OutDataType=sfix(16)  OutScaling=2^0
  Action Port : ActionPort  ActionType=case
  Out1 : Outport  OutDataType=sfix(16)  OutScaling=2^0
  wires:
  In1/1 -> Out1/1

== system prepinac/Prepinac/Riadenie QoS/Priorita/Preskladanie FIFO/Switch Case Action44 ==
  In1 : Inport  OutDataType=sfix(16)  OutScaling=2^0
  Action Port : ActionPort  ActionType=case
  Out1 : Outport  OutDataType=sfix(16)  OutScaling=2^0
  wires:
  In1/1 -> Out1/1

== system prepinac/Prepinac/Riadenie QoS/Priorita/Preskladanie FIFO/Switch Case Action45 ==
  In1 : Inport  OutDataType=sfix(16)  OutScaling=2^0
  Action Port : ActionPort  ActionType=case
  Out1 : Outport  OutDataType=sfix(16)  OutScaling=2^0
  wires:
  In1/1 -> Out1/1

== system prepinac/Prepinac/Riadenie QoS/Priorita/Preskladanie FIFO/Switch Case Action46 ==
  In1 : Inport  OutDataType=sfix(16)  OutScaling=2^0
  Action Port : ActionPort  ActionType=case
  Out1 : Outport  OutDataType=sfix(16)  OutScaling=2^0
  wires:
  In1/1 -> Out1/1

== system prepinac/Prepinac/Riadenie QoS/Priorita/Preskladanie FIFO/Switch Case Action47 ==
  In1 : Inport  OutDataType=sfix(16)  OutScaling=2^0
  Action Port : ActionPort  ActionType=case
  Out1 : Outport  OutDataType=sfix(16)  OutScaling=2^0
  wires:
  In1/1 -> Out1/1

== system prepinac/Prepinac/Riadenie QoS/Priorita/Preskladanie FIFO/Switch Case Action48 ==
  In1 : Inport  OutDataType=sfix(16)  OutScaling=2^0
  Action Port : ActionPort  ActionType=case
  Out1 : Outport  OutDataType=sfix(16)  OutScaling=2^0
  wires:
  In1/1 -> Out1/1

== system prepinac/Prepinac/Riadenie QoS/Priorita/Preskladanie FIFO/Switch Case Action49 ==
  In1 : Inport  OutDataType=sfix(16)  OutScaling=2^0
  Action Port : ActionPort  ActionType=case
  Out1 : Outport  OutDataType=sfix(16)  OutScaling=2^0
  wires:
  In1/1 -> Out1/1

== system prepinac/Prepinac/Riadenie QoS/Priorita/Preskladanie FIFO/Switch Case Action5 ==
  In1 : Inport  OutDataType=sfix(16)  OutScaling=2^0
  Action Port : ActionPort  ActionType=case
  Out1 : Outport  OutDataType=sfix(16)  OutScaling=2^0
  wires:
  In1/1 -> Out1/1

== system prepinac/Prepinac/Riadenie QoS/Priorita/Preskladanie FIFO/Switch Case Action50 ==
  In1 : Inport  OutDataType=sfix(16)  OutScaling=2^0
  Action Port : ActionPort  ActionType=case
  Out1 : Outport  OutDataType=sfix(16)  OutScaling=2^0
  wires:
  In1/1 -> Out1/1

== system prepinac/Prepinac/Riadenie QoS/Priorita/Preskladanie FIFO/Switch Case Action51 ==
  In1 : Inport  OutDataType=sfix(16)  OutScaling=2^0
  Action Port : ActionPort  ActionType=case
  Out1 : Outport  OutDataType=sfix(16)  OutScaling=2^0
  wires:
  In1/1 -> Out1/1

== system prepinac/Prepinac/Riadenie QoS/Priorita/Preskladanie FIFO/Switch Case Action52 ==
  In1 : Inport  OutDataType=sfix(16)  OutScaling=2^0
  Action Port : ActionPort  ActionType=case
  Out1 : Outport  OutDataType=sfix(16)  OutScaling=2^0
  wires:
  In1/1 -> Out1/1

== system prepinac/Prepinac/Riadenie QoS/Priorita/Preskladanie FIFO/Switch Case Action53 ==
  In1 : Inport  OutDataType=sfix(16)  OutScaling=2^0
  Action Port : ActionPort  ActionType=case
  Out1 : Outport  OutDataType=sfix(16)  OutScaling=2^0
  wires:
  In1/1 -> Out1/1

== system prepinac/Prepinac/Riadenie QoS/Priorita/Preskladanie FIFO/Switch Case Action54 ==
  In1 : Inport  OutDataType=sfix(16)  OutScaling=2^0
  Action Port : ActionPort  ActionType=case
  Out1 : Outport  OutDataType=sfix(16)  OutScaling=2^0
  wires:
  In1/1 -> Out1/1

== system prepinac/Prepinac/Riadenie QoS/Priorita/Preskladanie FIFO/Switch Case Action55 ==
  In1 : Inport  OutDataType=sfix(16)  OutScaling=2^0
  Action Port : ActionPort  ActionType=case
  Out1 : Outport  OutDataType=sfix(16)  OutScaling=2^0
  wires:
  In1/1 -> Out1/1

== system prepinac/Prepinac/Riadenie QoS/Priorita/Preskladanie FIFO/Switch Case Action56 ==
  In1 : Inport  OutDataType=sfix(16)  OutScaling=2^0
  Action Port : ActionPort  ActionType=case
  Out1 : Outport  OutDataType=sfix(16)  OutScaling=2^0
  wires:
  In1/1 -> Out1/1

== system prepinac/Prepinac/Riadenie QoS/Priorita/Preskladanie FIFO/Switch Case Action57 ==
  In1 : Inport  OutDataType=sfix(16)  OutScaling=2^0
  Action Port : ActionPort  ActionType=case
  Out1 : Outport  OutDataType=sfix(16)  OutScaling=2^0
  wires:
  In1/1 -> Out1/1

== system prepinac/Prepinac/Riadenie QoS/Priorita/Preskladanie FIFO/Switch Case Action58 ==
  In1 : Inport  OutDataType=sfix(16)  OutScaling=2^0
  Action Port : ActionPort  ActionType=case
  Out1 : Outport  OutDataType=sfix(16)  OutScaling=2^0
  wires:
  In1/1 -> Out1/1

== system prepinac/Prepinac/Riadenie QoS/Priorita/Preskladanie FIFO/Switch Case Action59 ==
  In1 : Inport  OutDataType=sfix(16)  OutScaling=2^0
  Action Port : ActionPort  ActionType=case
  Out1 : Outport  OutDataType=sfix(16)  OutScaling=2^0
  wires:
  In1/1 -> Out1/1

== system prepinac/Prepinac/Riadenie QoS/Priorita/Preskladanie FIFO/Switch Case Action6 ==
  In1 : Inport  OutDataType=sfix(16)  OutScaling=2^0
  Action Port : ActionPort  ActionType=case
  Out1 : Outport  OutDataType=sfix(16)  OutScaling=2^0
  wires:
  In1/1 -> Out1/1

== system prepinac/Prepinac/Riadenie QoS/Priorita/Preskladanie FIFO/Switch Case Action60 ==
  In1 : Inport  OutDataType=sfix(16)  OutScaling=2^0
  Action Port : ActionPort  ActionType=case
  Out1 : Outport  OutDataType=sfix(16)  OutScaling=2^0
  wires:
  In1/1 -> Out1/1

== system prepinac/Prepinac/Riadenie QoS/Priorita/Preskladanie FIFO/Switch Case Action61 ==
  In1 : Inport  OutDataType=sfix(16)  OutScaling=2^0
  Action Port : ActionPort  ActionType=case
  Out1 : Outport  OutDataType=sfix(16)  OutScaling=2^0
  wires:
  In1/1 -> Out1/1

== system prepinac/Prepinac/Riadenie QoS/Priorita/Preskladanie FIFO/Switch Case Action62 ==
  In1 : Inport  OutDataType=sfix(16)  OutScaling=2^0
  Action Port : ActionPort  ActionType=case
  Out1 : Outport  OutDataType=sfix(16)  OutScaling=2^0
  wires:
  In1/1 -> Out1/1

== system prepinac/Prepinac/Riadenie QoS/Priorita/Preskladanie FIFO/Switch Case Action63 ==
  In1 : Inport  OutDataType=sfix(16)  OutScaling=2^0
  Action Port : ActionPort  ActionType=case
  Out1 : Outport  OutDataType=sfix(16)  OutScaling=2^0
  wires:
  In1/1 -> Out1/1

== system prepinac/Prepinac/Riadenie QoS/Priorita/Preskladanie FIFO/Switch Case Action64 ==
  In1 : Inport  OutDataType=sfix(16)  OutScaling=2^0
  Action Port : ActionPort  ActionType=case
  Out1 : Outport  OutDataType=sfix(16)  OutScaling=2^0
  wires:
  In1/1 -> Out1/1

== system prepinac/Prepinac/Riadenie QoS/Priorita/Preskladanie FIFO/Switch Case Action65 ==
  In1 : Inport  OutDataType=sfix(16)  OutScaling=2^0
  Action Port : ActionPort  ActionType=case
  Out1 : Outport  OutDataType=sfix(16)  OutScaling=2^0
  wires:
  In1/1 -> Out1/1

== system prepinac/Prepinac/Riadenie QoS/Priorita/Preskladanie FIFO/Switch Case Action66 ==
  In1 : Inport  OutDataType=sfix(16)  OutScaling=2^0
  Action Port : ActionPort  ActionType=case
  Out1 : Outport  OutDataType=sfix(16)  OutScaling=2^0
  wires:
  In1/1 -> Out1/1

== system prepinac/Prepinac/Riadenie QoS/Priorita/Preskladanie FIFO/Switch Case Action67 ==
  In1 : Inport  OutDataType=sfix(16)  OutScaling=2^0
  Action Port : ActionPort  ActionType=case
  Out1 : Outport  OutDataType=sfix(16)  OutScaling=2^0
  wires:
  In1/1 -> Out1/1

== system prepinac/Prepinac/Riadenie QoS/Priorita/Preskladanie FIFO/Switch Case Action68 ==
  In1 : Inport  OutDataType=sfix(16)  OutScaling=2^0
  Action Port : ActionPort  ActionType=case
  Out1 : Outport  OutDataType=sfix(16)  OutScaling=2^0
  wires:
  In1/1 -> Out1/1

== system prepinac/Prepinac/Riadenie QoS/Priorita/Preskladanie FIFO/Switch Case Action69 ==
  In1 : Inport  OutDataType=sfix(16)  OutScaling=2^0
  Action Port : ActionPort  ActionType=case
  Out1 : Outport  OutDataType=sfix(16)  OutScaling=2^0
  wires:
  In1/1 -> Out1/1

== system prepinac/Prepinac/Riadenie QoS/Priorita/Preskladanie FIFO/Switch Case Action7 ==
  In1 : Inport  OutDataType=sfix(16)  OutScaling=2^0
  Action Port : ActionPort  ActionType=case
  Out1 : Outport  OutDataType=sfix(16)  OutScaling=2^0
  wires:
  In1/1 -> Out1/1

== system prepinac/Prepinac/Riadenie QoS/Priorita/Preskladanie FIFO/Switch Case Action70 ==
  In1 : Inport  OutDataType=sfix(16)  OutScaling=2^0
  Action Port : ActionPort  ActionType=case
  Out1 : Outport  OutDataType=sfix(16)  OutScaling=2^0
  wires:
  In1/1 -> Out1/1

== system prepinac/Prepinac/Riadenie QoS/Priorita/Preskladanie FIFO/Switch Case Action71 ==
  In1 : Inport  OutDataType=sfix(16)  OutScaling=2^0
  Action Port : ActionPort  ActionType=case
  Out1 : Outport  OutDataType=sfix(16)  OutScaling=2^0
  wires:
  In1/1 -> Out1/1

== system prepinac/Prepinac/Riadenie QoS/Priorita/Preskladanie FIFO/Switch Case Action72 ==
  In1 : Inport  OutDataType=sfix(16)  OutScaling=2^0
  Action Port : ActionPort  ActionType=case
  Out1 : Outport  OutDataType=sfix(16)  OutScaling=2^0
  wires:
  In1/1 -> Out1/1

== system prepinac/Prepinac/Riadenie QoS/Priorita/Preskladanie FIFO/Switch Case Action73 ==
  In1 : Inport  OutDataType=sfix(16)  OutScaling=2^0
  Action Port : ActionPort  ActionType=case
  Out1 : Outport  OutDataType=sfix(16)  OutScaling=2^0
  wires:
  In1/1 -> Out1/1

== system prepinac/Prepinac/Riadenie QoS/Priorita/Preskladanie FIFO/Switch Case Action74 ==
  In1 : Inport  OutDataType=sfix(16)  OutScaling=2^0
  Action Port : ActionPort  ActionType=case
  Out1 : Outport  OutDataType=sfix(16)  OutScaling=2^0
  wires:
  In1/1 -> Out1/1

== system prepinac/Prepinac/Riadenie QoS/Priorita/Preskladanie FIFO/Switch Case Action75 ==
  In1 : Inport  OutDataType=sfix(16)  OutScaling=2^0
  Action Port : ActionPort  ActionType=case
  Out1 : Outport  OutDataType=sfix(16)  OutScaling=2^0
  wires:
  In1/1 -> Out1/1

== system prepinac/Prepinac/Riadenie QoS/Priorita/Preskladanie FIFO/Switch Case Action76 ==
  In1 : Inport  OutDataType=sfix(16)  OutScaling=2^0
  Action Port : ActionPort  ActionType=case
  Out1 : Outport  OutDataType=sfix(16)  OutScaling=2^0
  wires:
  In1/1 -> Out1/1

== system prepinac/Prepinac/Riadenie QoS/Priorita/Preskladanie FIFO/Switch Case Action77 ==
  In1 : Inport  OutDataType=sfix(16)  OutScaling=2^0
  Action Port : ActionPort  ActionType=case
  Out1 : Outport  OutDataType=sfix(16)  OutScaling=2^0
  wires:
  In1/1 -> Out1/1

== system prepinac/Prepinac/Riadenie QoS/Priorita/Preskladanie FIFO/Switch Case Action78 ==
  In1 : Inport  OutDataType=sfix(16)  OutScaling=2^0
  Action Port : ActionPort  ActionType=case
  Out1 : Outport  OutDataType=sfix(16)  OutScaling=2^0
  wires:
  In1/1 -> Out1/1

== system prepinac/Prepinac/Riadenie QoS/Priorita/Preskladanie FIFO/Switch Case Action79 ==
  In1 : Inport  OutDataType=sfix(16)  OutScaling=2^0
  Action Port : ActionPort  ActionType=case
  Out1 : Outport  OutDataType=sfix(16)  OutScaling=2^0
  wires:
  In1/1 -> Out1/1

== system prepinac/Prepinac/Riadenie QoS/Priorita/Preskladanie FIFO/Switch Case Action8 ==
  In1 : Inport  OutDataType=sfix(16)  OutScaling=2^0
  Action Port : ActionPort  ActionType=case
  Out1 : Outport  OutDataType=sfix(16)  OutScaling=2^0
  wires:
  In1/1 -> Out1/1

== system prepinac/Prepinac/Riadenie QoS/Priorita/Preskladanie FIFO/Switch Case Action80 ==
  In1 : Inport  OutDataType=sfix(16)  OutScaling=2^0
  Action Port : ActionPort  ActionType=case
  Out1 : Outport  OutDataType=sfix(16)  OutScaling=2^0
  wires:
  In1/1 -> Out1/1

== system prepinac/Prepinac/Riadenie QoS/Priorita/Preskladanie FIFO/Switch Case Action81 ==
  In1 : Inport  OutDataType=sfix(16)  OutScaling=2^0
  Action Port : ActionPort  ActionType=case
  Out1 : Outport  OutDataType=sfix(16)  OutScaling=2^0
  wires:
  In1/1 -> Out1/1

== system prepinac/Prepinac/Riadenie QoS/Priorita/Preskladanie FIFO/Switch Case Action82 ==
  In1 : Inport  OutDataType=sfix(16)  OutScaling=2^0
  Action Port : ActionPort  ActionType=case
  Out1 : Outport  OutDataType=sfix(16)  OutScaling=2^0
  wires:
  In1/1 -> Out1/1

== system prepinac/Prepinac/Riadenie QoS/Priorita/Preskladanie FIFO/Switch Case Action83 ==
  In1 : Inport  OutDataType=sfix(16)  OutScaling=2^0
  Action Port : ActionPort  ActionType=case
  Out1 : Outport  OutDataType=sfix(16)  OutScaling=2^0
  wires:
  In1/1 -> Out1/1

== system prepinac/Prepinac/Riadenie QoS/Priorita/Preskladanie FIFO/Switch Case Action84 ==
  In1 : Inport  OutDataType=sfix(16)  OutScaling=2^0
  Action Port : ActionPort  ActionType=case
  Out1 : Outport  OutDataType=sfix(16)  OutScaling=2^0
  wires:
  In1/1 -> Out1/1

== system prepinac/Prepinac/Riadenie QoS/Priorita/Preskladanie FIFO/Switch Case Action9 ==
  In1 : Inport  OutDataType=sfix(16)  OutScaling=2^0
  Action Port : ActionPort  ActionType=case
  Out1 : Outport  OutDataType=sfix(16)  OutScaling=2^0
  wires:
  In1/1 -> Out1/1

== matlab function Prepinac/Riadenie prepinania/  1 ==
function y = prepinanie(MAC_prijata, MAC_arp)
if MAC_prijata==MAC_arp;
   y=2;
else
  y=1;
end;

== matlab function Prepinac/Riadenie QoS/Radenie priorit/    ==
function y = triedenie(x)
tmp=0; 
for j=1:3
for i=1:3
    if x(i)<x(i+1)
    else
       tmp=x(i);
        x(i)=x(i+1);
        x(i+1)=tmp;  
    end;
end;
end;
y=x;

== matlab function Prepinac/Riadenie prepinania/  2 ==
function y = prepinanie(MAC_prijata, MAC_arp)
if MAC_prijata==MAC_arp;
   y=2;
else
  y=1;
end;

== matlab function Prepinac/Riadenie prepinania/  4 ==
function y = prepinanie(MAC_prijata, MAC_arp)
if MAC_prijata==MAC_arp;
   y=2;
else
  y=1;
end;

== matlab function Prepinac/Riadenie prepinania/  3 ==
function y = prepinanie(MAC_prijata, MAC_arp)
if MAC_prijata==MAC_arp;
   y=2;
else
  y=1;
end;

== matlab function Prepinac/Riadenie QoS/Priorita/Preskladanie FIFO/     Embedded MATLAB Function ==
function y = zvysenie_priority(x)
for i=1:3
    for j=1:(4-i)
        if x(i)==x(i+j)
            x(i+j)=x(i+j)+1
        end;
    end;
end;
y=x;
